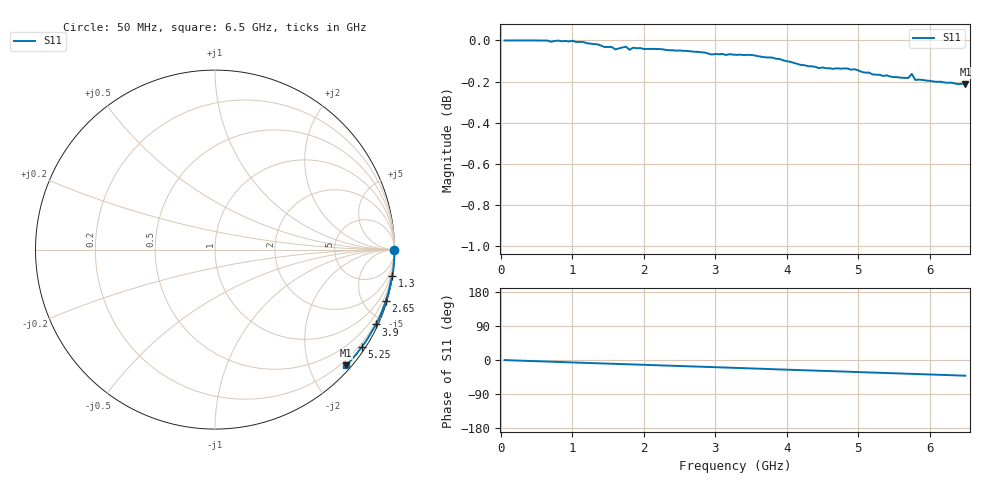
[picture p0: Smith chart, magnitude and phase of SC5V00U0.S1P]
! Infineon Technologies  Discrete & RF Semiconductors
! BAR63-02L
! Si PIN Diode in TSLP-2
! VR = 5 V
! S-Parameters:  March  2002
# GHz  S  MA  R  50
!  f  S11
! GHz  MAG  ANG
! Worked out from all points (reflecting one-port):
!   130 points, 50 MHz to 6.5 GHz, reference 50 ohm
!   lowest |S11| = -0.2 dB at 6.5 GHz (marker M1), VSWR 81.14, Z = 4.93 - j132 ohm
!   phase of S11 starts at -0 deg and turns -41 deg over the sweep
!   S11 on the Smith chart (normalised r, x): 50 MHz: open; 1.3 GHz: 0, -14; 2.65 GHz: 0.14, -6.77; 3.9 GHz: 0.11, -4.53; 5.25 GHz: 0.12, -3.33; 6.5 GHz: 0.10, -2.64
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0.05  1 -0.2
0.2  1 -1.3
0.55  0.9999 -3.5
0.6  0.9999 -3.9
0.85  0.9995 -5.4
0.9  0.9997 -5.8
1.3  0.998 -8.4
1.6  0.995 -10.2
1.7  0.9961 -10.8
1.75  0.9965 -11.2
1.8  0.9948 -11.5
2.1  0.9952 -13.3
2.15  0.9953 -13.7
2.5  0.9944 -15.9
2.65  0.9939 -16.8
2.7  0.9937 -17.2
3.3  0.992 -20.9
3.5  0.9919 -22.2
3.9  0.9897 -24.9
4.1  0.9875 -26.2
4.55  0.9846 -28.9
4.9  0.9838 -31.2
5.25  0.981 -33.4
5.7  0.9792 -36.3
5.75  0.9814 -36.5
5.8  0.9781 -36.9
6.15  0.9772 -39.1
6.5  0.9757 -41.4
